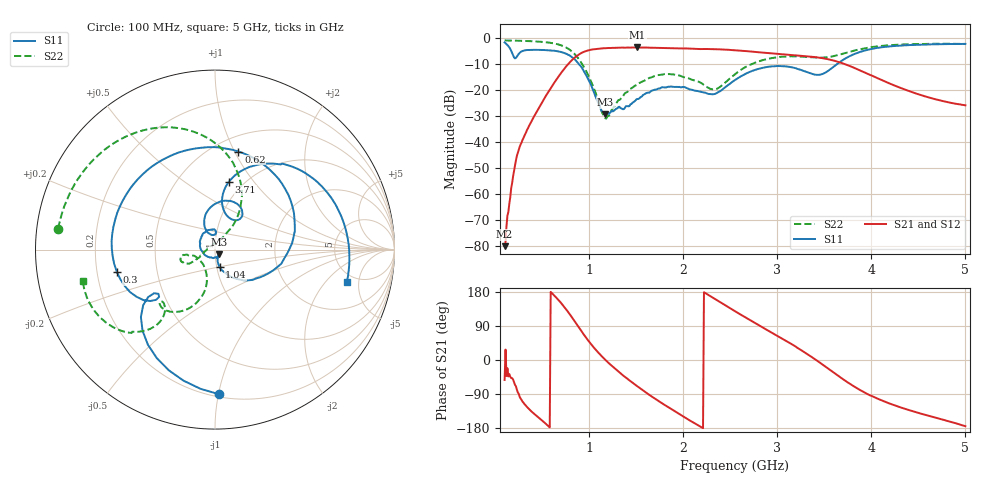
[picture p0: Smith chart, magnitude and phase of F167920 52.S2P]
!  2-Port S-parameters saved by WinCal
! VAR MeasName=S-Parameters (CALIBRATED_DATA) read from VNA (N5242A)
! VAR MeasDate=2016-11-22 9:58:05
! VAR NAME=F167920 52
! VAR FILENAME=F167920 52.S2P
! VAR DATE=2016-11-22 9:58:05
! VAR PHYS_PORTS=1,2
# Hz S DB R 50
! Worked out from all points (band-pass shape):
!   491 points, 100 MHz to 5 GHz, reference 50 ohm
!   highest |S21| = -3.76 dB at 1.51 GHz (marker M1); lowest = -80.0 dB at 100 MHz (marker M2)
!   |S21| within 3 dB of the highest: 878.4 MHz to 3.185 GHz (2.307 GHz wide, 114 % of centre)
!   lowest |S11| = -29.4 dB at 1.17 GHz (marker M3), VSWR 1.07, Z = 52 - j2.78 ohm
!   |S11| at or under -10 dB: 886.6 MHz to 3.64 GHz (2.754 GHz wide, 122 % of centre)
!   |S22| runs from -31.1 to -1.1 dB; largest |S21 - S12| = 0.0015
!   S11 on the Smith chart (normalised r, x): 100 MHz: 0.22, -1.01; 300 MHz: 0.28, -0.10; 620 MHz: 0.65, +1.04; 1.04 GHz: 1.03, -0.20; 3.71 GHz: 0.86, +0.76; 5 GHz: 4.14, -3.50
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1e8  -1.86 -88.2  -79.97 -52.7  -81.20 -58.6  -1.10 172.4
1.6e8  -4.35 -131.8  -61.29 -44.0  -59.74 -46.2  -1.14 167.8
2.1e8  -7.96 -142.0  -49.06 -65.4  -49.07 -62.7  -1.17 163.9
3e8  -5.02 -167.3  -38.55 -112.5  -38.57 -112.2  -1.26 156.6
4.7e8  -4.71 127.4  -26.57 -153.7  -26.58 -153.7  -1.56 140.4
6.2e8  -5.01 76.6  -17.75 172.3  -17.75 172.3  -2.20 121.2
7.7e8  -6.48 21.1  -10.41 128.5  -10.41 128.6  -4.12 93.7
9.2e8  -11.42 -39.0  -5.83 75.3  -5.82 75.3  -9.91 62.2
1.04e9  -20.09 -75.3  -4.52 35.4  -4.51 35.4  -18.55 54.3
1.17e9  -29.42 -52.1  -4.07 0.7  -4.07 0.7  -30.93 118.3
1.51e9  -23.55 -158.8  -3.76 -69.1  -3.77 -69.1  -18.06 -151.4
1.74e9  -19.50 133.2  -3.97 -108.6  -3.97 -108.6  -14.34 -157.8
2.12e9  -20.34 87.1  -4.32 -167.2  -4.32 -167.2  -16.41 -167.7
2.34e9  -21.55 102.7  -4.46 160.4  -4.46 160.4  -19.73 -135.5
2.55e9  -16.26 112.9  -4.85 128.8  -4.85 128.7  -14.00 -103.7
2.91e9  -11.16 79.5  -6.00 76.4  -6.01 76.4  -8.08 -119.3
3.37e9  -13.93 54.5  -7.36 7.1  -7.37 7.3  -7.58 -136.5
3.49e9  -13.81 72.1  -7.95 -13.6  -7.96 -13.5  -7.66 -133.4
3.71e9  -8.30 78.5  -10.06 -52.7  -10.08 -52.5  -6.04 -127.3
3.93e9  -4.96 58.1  -13.37 -86.2  -13.41 -86.0  -4.11 -132.8
4.19e9  -3.39 35.4  -17.53 -114.6  -17.56 -114.1  -2.93 -142.7
5e9  -2.43 -13.9  -25.96 -174.7  -25.95 -174.4  -2.44 -166.8
